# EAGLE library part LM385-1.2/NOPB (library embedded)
Voltage Ref LM385M Texas Instruments
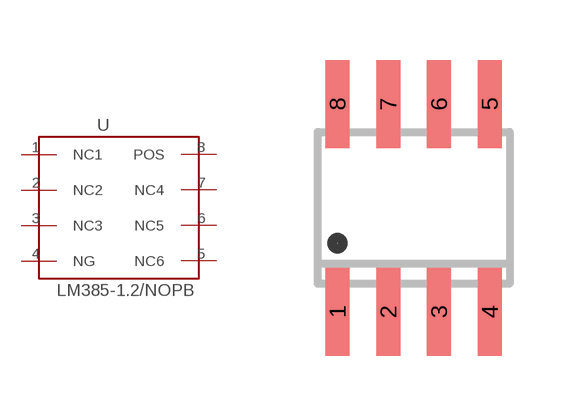
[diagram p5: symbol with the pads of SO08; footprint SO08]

Designator prefix U

## LM385-1.2/NOPB (DATASHEET: http://www.ti.com/lit/ds/symlink/lm385-1.2-n.pdf; DESCR: Voltage References Fixed 1.235 MicroPwr Vtg Ref - SOIC-8; FARNELL_NO: 2782470; MF: Texas Instruments; MF_PN: LM385MX-1.2/NOPB; PACKAGE: SOIC-8; PURCHASE: https://de.farnell.com/texas-instruments/lm385mx-1-2-nopb/spannungsreferenz-shunt-1-235v/dp/2782470; UNIT_PRICE: 0.60)  [SO08]
1  NC1  nc
2  NC2  nc
3  NC3  nc
4  NG
5  NC6  nc
6  NC5  nc
7  NC4  nc
8  POS

## Footprint SO08 (pad centres in mm)
Small Outline Package 8 NS Package M08A
smd 0.6 x 2.2: 1 -1.905,-2.6; 2 -0.635,-2.6; 3 0.635,-2.6; 4 1.905,-2.6; 5 1.905,2.6; 6 0.635,2.6; 7 -0.635,2.6; 8 -1.905,2.6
